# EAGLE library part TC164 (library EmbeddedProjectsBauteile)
SMD Widerstandsnetzwerk
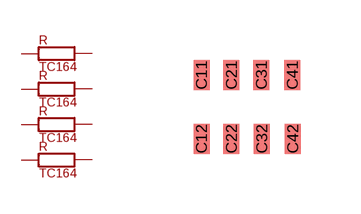
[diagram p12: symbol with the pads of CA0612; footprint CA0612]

Designator prefix R; gates G$1=TC1641 G$2=TC1641 G$3=TC1641 G$4=TC1641

## TC164  [CA0612]
C11  G$1:11
C12  G$1:12
C21  G$2:11
C22  G$2:12
C31  G$3:11
C32  G$3:12
C41  G$4:11
C42  G$4:12

## Footprint CA0612 (pad centres in mm)
smd 0.4 x 0.762: C11 -1.124,0.8; C12 -1.124,-0.8; C21 -0.375,0.8; C22 -0.375,-0.8; C31 0.375,0.8; C32 0.385,-0.8; C41 1.149,0.8; C42 1.159,-0.8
